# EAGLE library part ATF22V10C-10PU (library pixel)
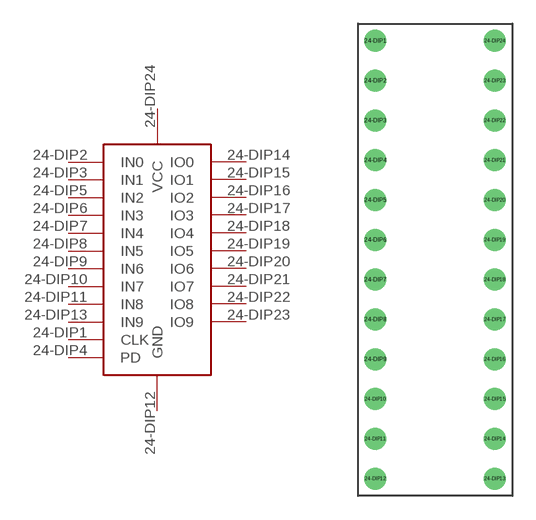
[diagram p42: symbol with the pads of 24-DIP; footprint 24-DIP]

Designator prefix -

## ATF22V10C-10PU  [24-DIP]
24-DIP1  CLK
24-DIP2  IN0
24-DIP3  IN1
24-DIP4  PD
24-DIP5  IN2
24-DIP6  IN3
24-DIP7  IN4
24-DIP8  IN5
24-DIP9  IN6
24-DIP10  IN7
24-DIP11  IN8
24-DIP12  GND
24-DIP13  IN9
24-DIP14  IO0
24-DIP15  IO1
24-DIP16  IO2
24-DIP17  IO3
24-DIP18  IO4
24-DIP19  IO5
24-DIP20  IO6
24-DIP21  IO7
24-DIP22  IO8
24-DIP23  IO9
24-DIP24  VCC

## Footprint 24-DIP (pad centres in mm)
drill 0.9: 24-DIP1 -3.81,13.97; 24-DIP2 -3.81,11.43; 24-DIP3 -3.81,8.89; 24-DIP4 -3.81,6.35; 24-DIP5 -3.81,3.81; 24-DIP6 -3.81,1.27; 24-DIP7 -3.81,-1.27; 24-DIP8 -3.81,-3.81; 24-DIP9 -3.81,-6.35; 24-DIP10 -3.81,-8.89; 24-DIP11 -3.81,-11.43; 24-DIP12 -3.81,-13.97; 24-DIP13 3.81,-13.97; 24-DIP14 3.81,-11.43; 24-DIP15 3.81,-8.89; 24-DIP16 3.81,-6.35; 24-DIP17 3.81,-3.81; 24-DIP18 3.81,-1.27; 24-DIP19 3.81,1.27; 24-DIP20 3.81,3.81; 24-DIP21 3.81,6.35; 24-DIP22 3.81,8.89; 24-DIP23 3.81,11.43; 24-DIP24 3.81,13.97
